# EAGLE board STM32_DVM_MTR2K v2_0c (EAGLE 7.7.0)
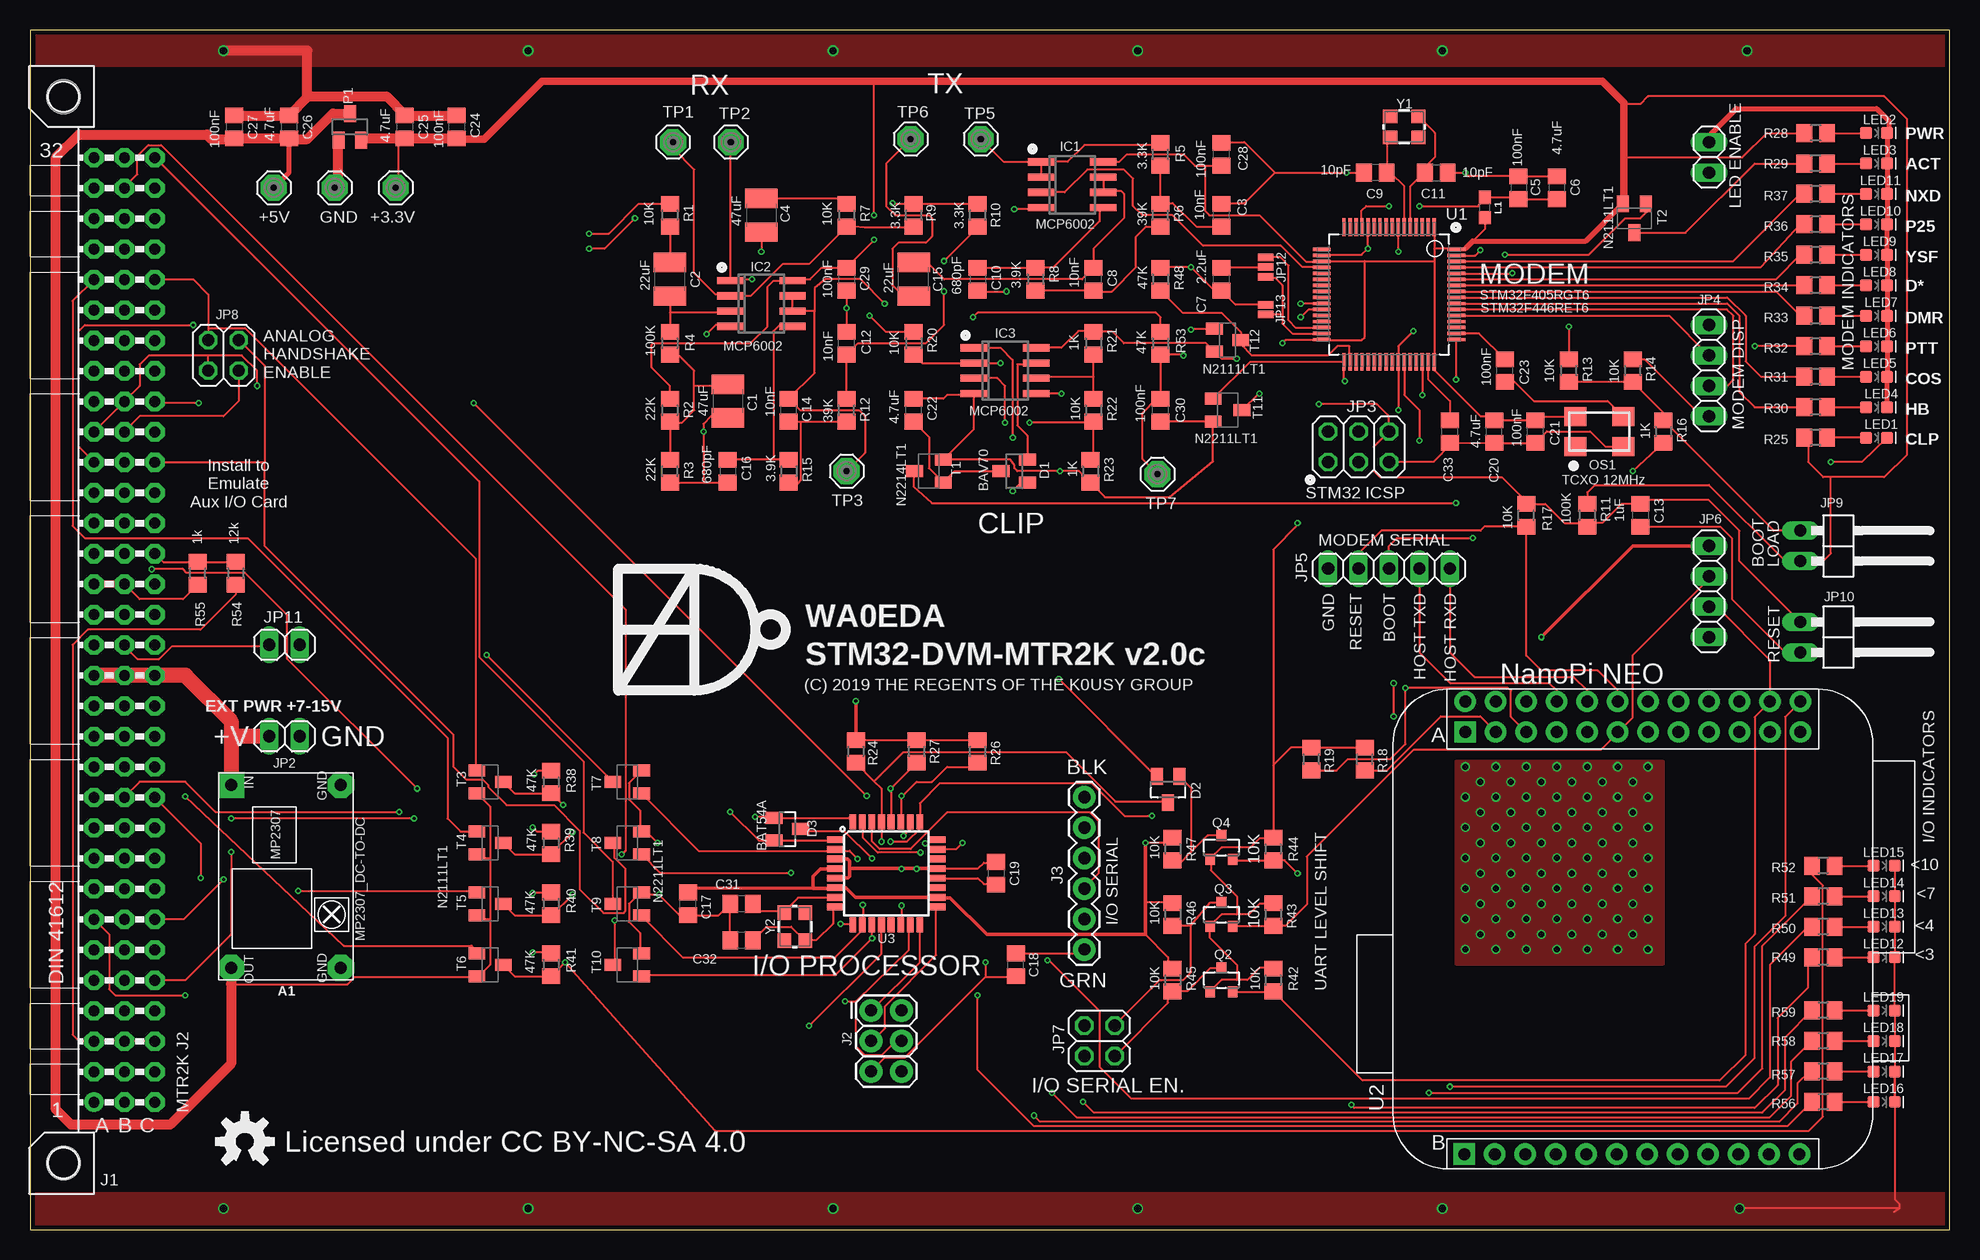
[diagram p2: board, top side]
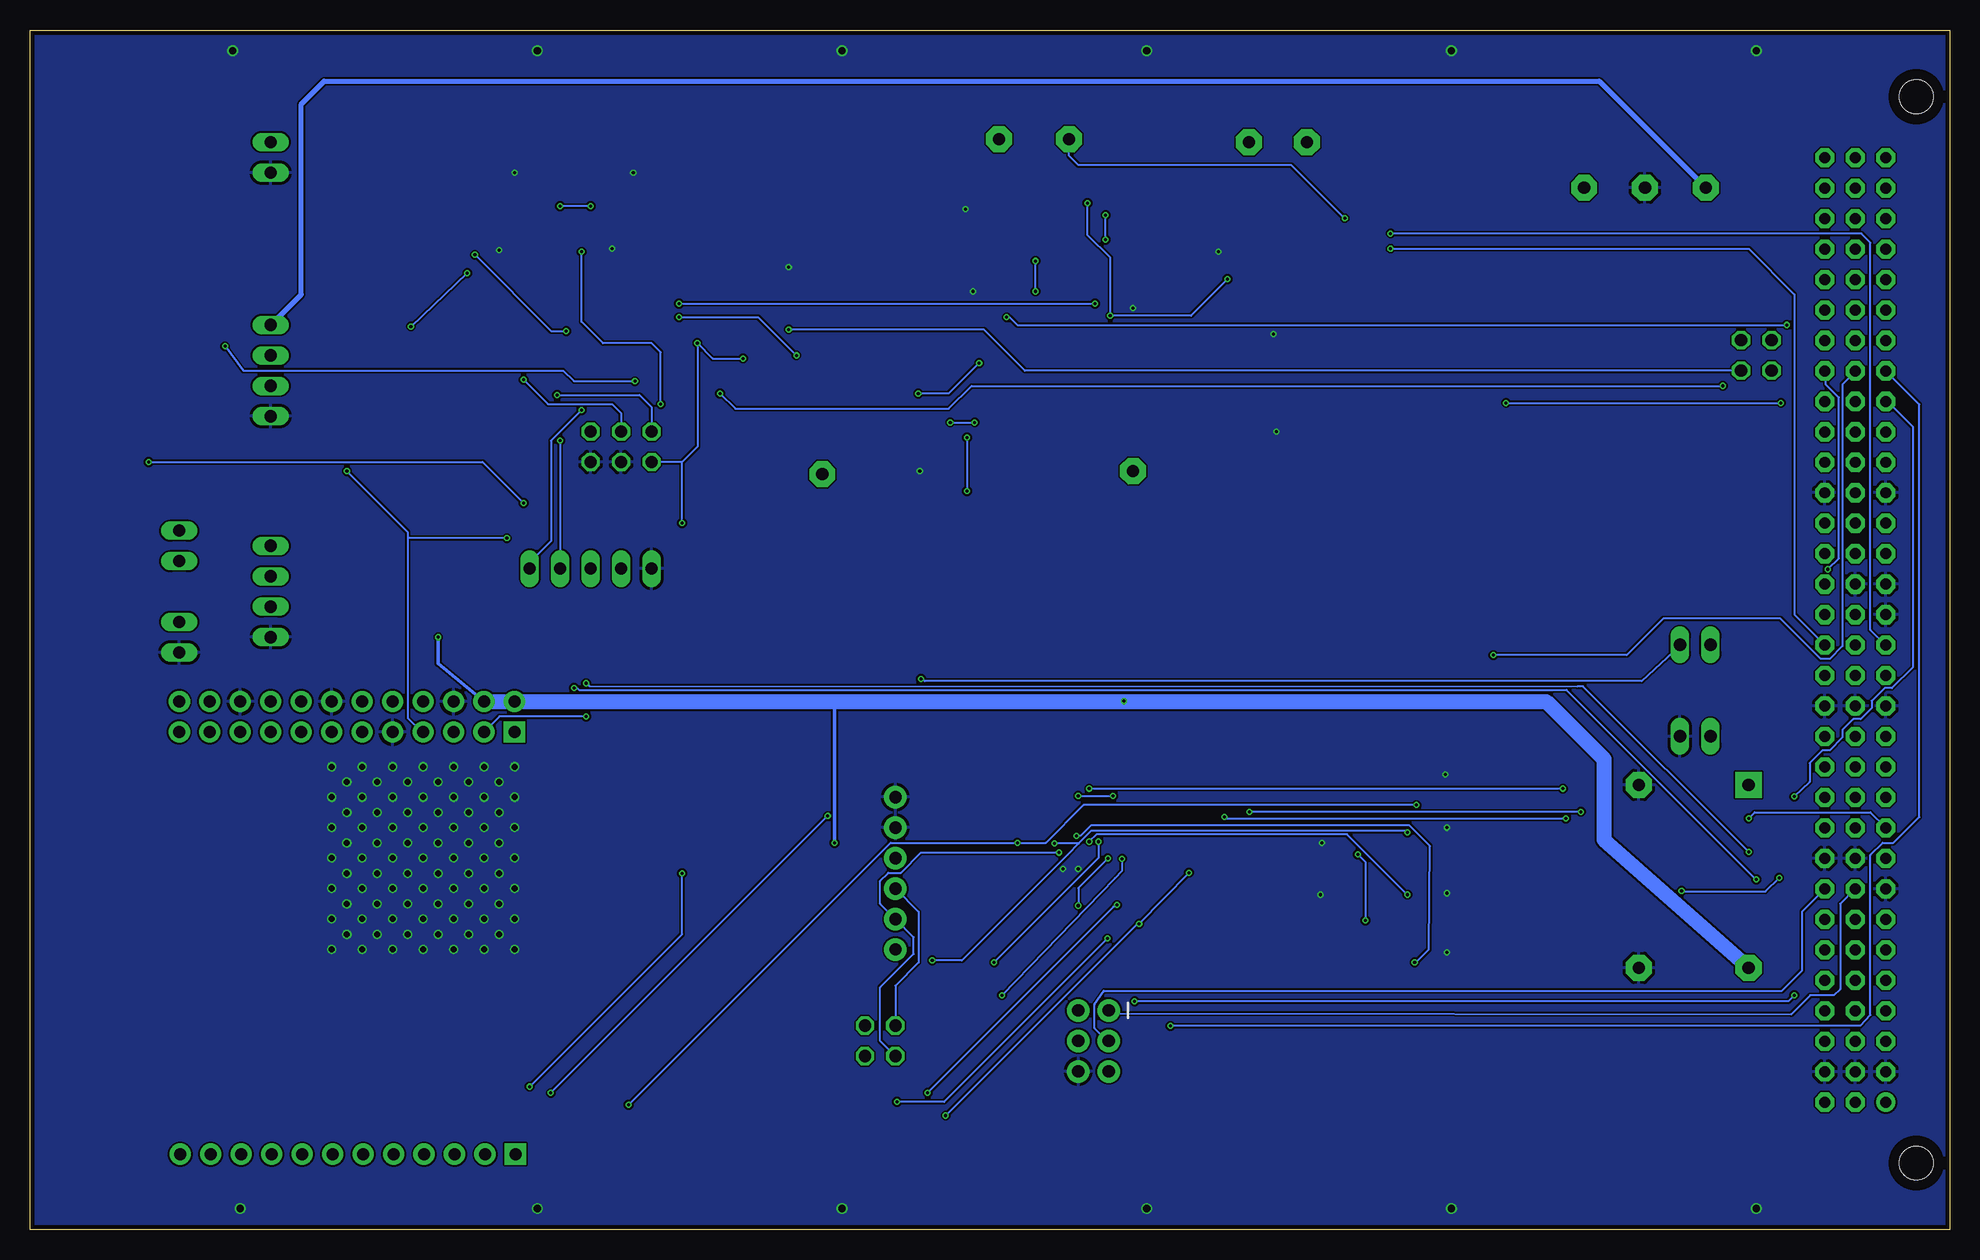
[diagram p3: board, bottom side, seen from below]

Size 160.02 x 100.03 mm. Coordinates in mm from the lower left corner, seen from the top.
Copper layers (1*16): Top 0.035559375mm / dielectric 1.6mm / Bottom 0.035559375mm
Design rules "oshpark-2layer-tented": minimum track width 6mil, minimum drill 10mil, track to track 6mil, track to pad 6mil, pad to pad 6mil, via to via 6mil, smd to smd 6mil, copper to edge 15mil, drill to drill 6mil, minimum pad ring 5mil, minimum via ring 5mil, stop-mask expansion 2.5mil, vias tented up to drill 20mil, thermal gap 10mil

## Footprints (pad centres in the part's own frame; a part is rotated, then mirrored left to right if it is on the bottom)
MCS10B = drill 1.016 pad 2.159 octagon: MP 0,0
MPS2307_DC-TO-DC = drill 1.016 pad 2.184 octagon: GND1 -7.62,4.572; GND2 7.62,4.572; OUT 7.62,-4.572 | drill 1.016 pad 2.184 square: IN -7.62,-4.572
C1210 = smd 1.6 x 2.7: 1 -1.4,0; 2 1.4,0
C0805 = smd 1.3 x 1.5: 1 -0.95,0; 2 0.95,0
SOT23C = smd 1 x 1.4: 1 -0.95,-1.1; 2 0.95,-1.1; 3 0,1.1
SOT23 = smd 1 x 1.4: 1 -0.95,-1.1; 2 0.95,-1.1; 3 0,1.1
SO08 = smd 0.6 x 2.2: 1 -1.905,-2.6; 2 -0.635,-2.6; 3 0.635,-2.6; 4 1.905,-2.6; 5 1.905,2.6; 6 0.635,2.6; 7 -0.635,2.6; 8 -1.905,2.6
VG96 = drill 0.914 pad 1.6: A1 154.94,39.37 | drill 0.914 pad 1.6 octagon: A2 154.94,36.83; A3 154.94,34.29; A4 154.94,31.75; A5 154.94,29.21; A6 154.94,26.67; A7 154.94,24.13; A8 154.94,21.59; A9 154.94,19.05; A10 154.94,16.51; A11 154.94,13.97; A12 154.94,11.43; A13 154.94,8.89; A14 154.94,6.35; A15 154.94,3.81; A16 154.94,1.27; A17 154.94,-1.27; A18 154.94,-3.81; A19 154.94,-6.35; A20 154.94,-8.89; A21 154.94,-11.43; A22 154.94,-13.97; A23 154.94,-16.51; A24 154.94,-19.05; A25 154.94,-21.59; A26 154.94,-24.13; A27 154.94,-26.67; A28 154.94,-29.21; A29 154.94,-31.75; A30 154.94,-34.29; A31 154.94,-36.83; A32 154.94,-39.37; B1 152.4,39.37; B2 152.4,36.83; B3 152.4,34.29; B4 152.4,31.75; B5 152.4,29.21; B6 152.4,26.67; B7 152.4,24.13; B8 152.4,21.59; B9 152.4,19.05; B10 152.4,16.51; B11 152.4,13.97; B12 152.4,11.43; B13 152.4,8.89; B14 152.4,6.35; B15 152.4,3.81; B16 152.4,1.27; B17 152.4,-1.27; B18 152.4,-3.81; B19 152.4,-6.35; B20 152.4,-8.89; B21 152.4,-11.43; B22 152.4,-13.97; B23 152.4,-16.51; B24 152.4,-19.05; B25 152.4,-21.59; B26 152.4,-24.13; B27 152.4,-26.67; B28 152.4,-29.21; B29 152.4,-31.75; B30 152.4,-34.29; B31 152.4,-36.83; B32 152.4,-39.37; C1 149.86,39.37; C2 149.86,36.83; C3 149.86,34.29; C4 149.86,31.75; C5 149.86,29.21; C6 149.86,26.67; C7 149.86,24.13; C8 149.86,21.59; C9 149.86,19.05; C10 149.86,16.51; C11 149.86,13.97; C12 149.86,11.43; C13 149.86,8.89; C14 149.86,6.35; C15 149.86,3.81; C16 149.86,1.27; C17 149.86,-1.27; C18 149.86,-3.81; C19 149.86,-6.35; C20 149.86,-8.89; C21 149.86,-11.43; C22 149.86,-13.97; C23 149.86,-16.51; C24 149.86,-19.05; C25 149.86,-21.59; C26 149.86,-24.13; C27 149.86,-26.67; C28 149.86,-29.21; C29 149.86,-31.75; C30 149.86,-34.29; C31 149.86,-36.83; C32 149.86,-39.37 | hole 2.794: 157.48,44.45; 157.48,-44.45
2X3 = drill 1.016 pad 1.88: 1 0,0; 2 0,2.54; 3 2.54,0; 4 2.54,2.54; 5 5.08,0; 6 5.08,2.54
FTDI_BASIC = drill 1.016 pad 1.88: CTS 10.16,0; DTR 0,0; GND 12.7,0; RXI 2.54,0; TXO 5.08,0; VCC 7.62,0
1X02 = drill 1.016 long: 1 -1.27,0; 2 1.27,0
2X03 = drill 1.016 octagon: 1 -2.54,-1.27; 2 -2.54,1.27; 3 0,-1.27; 4 0,1.27; 5 2.54,-1.27; 6 2.54,1.27
1X04 = drill 1.016 long: 1 -3.81,0; 2 -1.27,0; 3 1.27,0; 4 3.81,0
1X05 = drill 1.016 long: 1 -5.08,0; 2 -2.54,0; 3 0,0; 4 2.54,0; 5 5.08,0
2X02 = drill 1.016 octagon: 1 -1.27,-1.27; 2 -1.27,1.27; 3 1.27,-1.27; 4 1.27,1.27
1X02/90 = drill 1.016 long: 1 -1.27,-3.81; 2 1.27,-3.81
SMT-JUMPER_3_NO_NO-SILK = smd 0.635 x 1.27: 1 -0.813,0; 2 0,0; 3 0.813,0
SMT-JUMPER_2_NO_NO-SILK = smd 0.635 x 1.27: 1 -0.406,0; 2 0.406,0
0603 = smd 1.1 x 1: 1 -0.85,0; 2 0.85,0
LED-0603 = smd 1 x 1: A -0.877,0; C 0.877,0
5.2X3.4-4-PAD = smd 1.8 x 1.6: 1 -2,-1.25; 2 2,-1.25; 3 2,1.25; 4 -2,1.25
XC6206_SOT-23 = smd 1 x 1.4: 1 -0.95,-1.1; 2 0.95,-1.1; 3 0,1.1
SOT23' = smd 0.8 x 0.9: 1 -0.95,-1; 2 0.95,-1; 3 0,1
R0805 = smd 1.3 x 1.5: 1 -0.95,0; 2 0.95,0
SC59-BEC = smd 1 x 1.4: B -0.95,-1.2; C 0,1.2; E 0.95,-1.2
SOT23-BEC = smd 1 x 1.4: B -0.95,-1.1; C 0,1.1; E 0.95,-1.1
QFP50P1200X1200X160-64N = smd 1.473 x 0.279: 1 -5.613,3.759; 2 -5.613,3.251; 3 -5.613,2.743; 4 -5.613,2.261; 5 -5.613,1.753; 6 -5.613,1.245; 7 -5.613,0.762; 8 -5.613,0.254; 9 -5.613,-0.254; 10 -5.613,-0.762; 11 -5.613,-1.245; 12 -5.613,-1.753; 13 -5.613,-2.261; 14 -5.613,-2.743; 15 -5.613,-3.251; 16 -5.613,-3.759; 33 5.613,-3.759; 34 5.613,-3.251; 35 5.613,-2.743; 36 5.613,-2.261; 37 5.613,-1.753; 38 5.613,-1.245; 39 5.613,-0.762; 40 5.613,-0.254; 41 5.613,0.254; 42 5.613,0.762; 43 5.613,1.245; 44 5.613,1.753; 45 5.613,2.261; 46 5.613,2.743; 47 5.613,3.251; 48 5.613,3.759 | smd 0.279 x 1.473: 17 -3.759,-5.613; 18 -3.251,-5.613; 19 -2.743,-5.613; 20 -2.261,-5.613; 21 -1.753,-5.613; 22 -1.245,-5.613; 23 -0.762,-5.613; 24 -0.254,-5.613; 25 0.254,-5.613; 26 0.762,-5.613; 27 1.245,-5.613; 28 1.753,-5.613; 29 2.261,-5.613; 30 2.743,-5.613; 31 3.251,-5.613; 32 3.759,-5.613; 49 3.759,5.613; 50 3.251,5.613; 51 2.743,5.613; 52 2.261,5.613; 53 1.753,5.613; 54 1.245,5.613; 55 0.762,5.613; 56 0.254,5.613; 57 -0.254,5.613; 58 -0.762,5.613; 59 -1.245,5.613; 60 -1.753,5.613; 61 -2.261,5.613; 62 -2.743,5.613; 63 -3.251,5.613; 64 -3.759,5.613
NANOPI-NEO = drill 1 pad 1.778 square: A1 6.02,36.42; B1 5.94,1.227 | drill 1 pad 1.778: A2 6.02,38.96; A3 8.56,36.42; A4 8.56,38.96; A5 11.1,36.42; A6 11.1,38.96; A7 13.64,36.42; A8 13.64,38.96; A9 16.18,36.42; A10 16.18,38.96; A11 18.72,36.42; A12 18.72,38.96; A13 21.26,36.42; A14 21.26,38.96; A15 23.8,36.42; A16 23.8,38.96; A17 26.34,36.42; A18 26.34,38.96; A19 28.88,36.42; A20 28.88,38.96; A21 31.42,36.42; A22 31.42,38.96; A23 33.96,36.42; A24 33.96,38.96; B2 8.48,1.227; B3 11.02,1.227; B4 13.56,1.227; B5 16.1,1.227; B6 18.64,1.227; B7 21.18,1.227; B8 23.72,1.227; B9 26.26,1.227; B10 28.8,1.227; B11 31.34,1.227; B12 33.88,1.227
TQFP32-08 = smd 1.27 x 0.559: 1 -4.293,2.8; 2 -4.293,2; 3 -4.293,1.2; 4 -4.293,0.4; 5 -4.293,-0.4; 6 -4.293,-1.2; 7 -4.293,-2; 8 -4.293,-2.8; 17 4.293,-2.8; 18 4.293,-2; 19 4.293,-1.2; 20 4.293,-0.4; 21 4.293,0.4; 22 4.293,1.2; 23 4.293,2; 24 4.293,2.8 | smd 0.559 x 1.27: 9 -2.8,-4.293; 10 -2,-4.293; 11 -1.2,-4.293; 12 -0.4,-4.293; 13 0.4,-4.293; 14 1.2,-4.293; 15 2,-4.293; 16 2.8,-4.293; 25 2.8,4.293; 26 2,4.293; 27 1.2,4.293; 28 0.4,4.293; 29 -0.4,4.293; 30 -1.2,4.293; 31 -2,4.293; 32 -2.8,4.293
CRYSTAL-SMD-3.2X2.5MM = smd 1.2 x 1.1: 1 -1.175,-0.875; 2 1.175,-0.875; 3 1.175,0.875; 4 -1.175,0.875

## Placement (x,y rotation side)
+3.3V  MCS10B  [MCS10B]  30.48,86.87 0 top
+5V  MCS10B  [MCS10B]  20.32,86.87 0 top
A1  MP2307_DC-TO-DC  [MPS2307_DC-TO-DC]  21.34,29.46 270 top
C1  47uF  [C1210]  58.17,69.09 270 top
C2  22uF  [C1210]  53.34,79.25 90 top
C3  10nF  [C0805]  99.31,84.58 90 top
C4  47uF  [C1210]  60.96,84.58 270 top
C5  100nF  [C0805]  124.08,86.87 270 top
C6  4.7uF  [C0805]  127.25,86.87 270 top
C7  2.2uF  [C0805]  99.31,79.25 90 top
C8  10nF  [C0805]  88.65,79.25 90 top
C9  10pF  [C0805]  112.14,88.14 180 top
C10  680pF  [C0805]  78.99,79.25 270 top
C11  10pF  [C0805]  117.22,88.14 0 top
C12  10nF  [C0805]  68.07,73.91 90 top
C13  1uF  [C0805]  134.24,59.56 270 top
C14  10nF  [C0805]  63.25,68.33 90 top
C15  22uF  [C1210]  73.66,79.25 90 top
C16  680pF  [C0805]  58.17,63.25 270 top
C17  100nF  [C0805]  54.86,27.18 90 top
C18  100nF  [C0805]  82.17,22.1 90 top
C19  100nF  [C0805]  80.52,29.72 270 top
C20  4.7uF  [C0805]  122.05,66.55 90 top
C21  100nF  [C0805]  125.48,66.55 90 top
C22  4.7uF  [C0805]  73.66,68.33 90 top
C23  100nF  [C0805]  122.94,71.63 90 top
C24  100nF  [C0805]  35.56,91.95 270 top
C25  4.7uF  [C0805]  31.24,91.95 270 top
C26  4.7uF  [C0805]  21.59,91.95 270 top
C27  100nF  [C0805]  17.02,91.95 270 top
C28  100nF  [C0805]  99.31,89.66 90 top
C29  100nF  [C0805]  68.07,79.25 270 top
C30  100nF  [C0805]  94.23,68.33 90 top
C31  10pF  [C0805]  59.31,27.18 180 top
C32  10pF  [C0805]  59.31,24.13 180 top
C33  2.2uF  [C0805]  118.36,66.55 90 top
D1  BAV70  [SOT23C]  82.04,63.25 90 top
D2  BAT54A  [SOT23]  94.87,36.7 180 top
D3  BAT54A  [SOT23]  63.12,33.4 270 top
GND  MCS10B  [MCS10B]  25.4,86.87 0 top
IC1  MCP6002  [SO08]  86.87,87.12 270 top
IC2  MCP6002  [SO08]  60.96,77.22 270 top
IC3  MCP6002  [SO08]  81.28,71.63 270 top
J1  MTR2K J2  [VG96]  160.27,50.01 180 top
J2  AVR_SPI_ICSP  [2X3]  70.1,18.29 270 top
J3  I/O SERIAL  [FTDI_BASIC]  87.88,23.37 90 top
JP1  LED ENABLE  [1X02]  139.95,89.41 270 top
JP2  EXT PWR +7-15V  [1X02]  21.21,41.15 0 top
JP3  STM32 ICSP  [2X03]  110.74,65.28 0 top
JP4  MODEM DISP  [1X04]  139.95,71.63 270 top
JP5  MODEM SERIAL  [1X05]  113.28,55.12 180 top
JP6  SBC DISP  [1X04]  139.95,53.21 270 top
JP7  I/O SERIAL EN.  [2X02]  89.15,15.75 90 top
JP8  ANALOG HANDSHAKE ENABLE  [2X02]  16.13,72.9 180 top
JP9  BOOT  [1X02/90]  151.38,57.02 270 top
JP10  RESET  [1X02/90]  151.38,49.4 270 top
JP11  AVR RESET  [1X02]  21.21,48.77 0 top
JP12  405/446  [SMT-JUMPER_3_NO_NO-SILK]  103,80.26 270 top
JP13  446  [SMT-JUMPER_2_NO_NO-SILK]  103,76.71 90 top
L1  120Ω/100M  [0603]  121.28,85.22 90 top
LED1  RED  [LED-0603]  153.92,66.04 0 top
LED2  BLU  [LED-0603]  153.92,91.44 0 top
LED3  ORG  [LED-0603]  153.92,88.9 0 top
LED4  ORG  [LED-0603]  153.92,68.58 0 top
LED5  GRN  [LED-0603]  153.92,71.12 0 top
LED6  RED  [LED-0603]  153.92,73.66 0 top
LED7  YEL  [LED-0603]  153.92,76.2 0 top
LED8  YEL  [LED-0603]  153.92,78.74 0 top
LED9  YEL  [LED-0603]  153.92,81.28 0 top
LED10  YEL  [LED-0603]  153.92,83.82 0 top
LED11  YEL  [LED-0603]  153.92,86.36 0 top
LED12  GRN  [LED-0603]  154.56,22.73 0 top
LED13  GRN  [LED-0603]  154.56,25.27 0 top
LED14  GRN  [LED-0603]  154.56,27.81 0 top
LED15  GRN  [LED-0603]  154.56,30.35 0 top
LED16  RED  [LED-0603]  154.56,10.67 0 top
LED17  RED  [LED-0603]  154.56,13.21 0 top
LED18  RED  [LED-0603]  154.56,15.75 0 top
LED19  RED  [LED-0603]  154.56,18.29 0 top
OS1  TCXO 12MHz  [5.2X3.4-4-PAD]  130.81,66.55 0 top
P1  XC6206P332MR  [XC6206_SOT-23]  26.67,91.95 0 top
Q2  BSS138  [SOT23']  99.31,20.83 0 top
Q3  BSS138  [SOT23']  99.31,26.29 0 top
Q4  BSS138  [SOT23']  99.31,31.88 0 top
R1  10K  [R0805]  53.34,84.58 270 top
R2  22K  [R0805]  53.34,68.33 270 top
R3  22K  [R0805]  53.34,63.25 90 top
R4  100K  [R0805]  53.34,73.91 270 top
R5  3.3K  [R0805]  94.23,89.66 90 top
R6  39K  [R0805]  94.23,84.58 90 top
R7  10K  [R0805]  68.07,84.58 270 top
R8  3.9K  [R0805]  83.82,79.25 270 top
R9  3.3K  [R0805]  73.66,84.58 90 top
R10  3.3K  [R0805]  78.99,84.58 90 top
R11  100K  [R0805]  129.79,59.56 270 top
R12  39K  [R0805]  68.07,68.33 90 top
R13  10K  [R0805]  128.27,71.63 90 top
R14  10K  [R0805]  133.6,71.63 90 top
R15  3.9K  [R0805]  63.25,63.25 270 top
R16  1K  [R0805]  136.14,66.55 270 top
R17  10K  [R0805]  124.71,59.56 90 top
R18  3.3K  [R0805]  111.25,39.24 90 top
R19  3.3K  [R0805]  106.81,39.24 90 top
R20  10K  [R0805]  73.66,73.91 270 top
R21  1K  [R0805]  88.65,73.91 270 top
R22  10K  [R0805]  88.65,68.33 270 top
R23  1K  [R0805]  88.39,63.25 270 top
R24  10K  [R0805]  68.83,39.88 270 top
R25  560  [R0805]  148.84,66.04 180 top
R26  3.3K  [R0805]  78.99,39.88 90 top
R27  3.3K  [R0805]  73.91,39.88 90 top
R28  1K  [R0805]  148.84,91.44 180 top
R29  560  [R0805]  148.84,88.9 180 top
R30  560  [R0805]  148.84,68.58 180 top
R31  1K  [R0805]  148.84,71.12 180 top
R32  560  [R0805]  148.84,73.66 180 top
R33  560  [R0805]  148.84,76.2 180 top
R34  560  [R0805]  148.84,78.74 180 top
R35  560  [R0805]  148.84,81.28 180 top
R36  560  [R0805]  148.84,83.82 180 top
R37  560  [R0805]  148.84,86.36 180 top
R38  47K  [R0805]  43.43,37.34 270 top
R39  47K  [R0805]  43.43,32.26 270 top
R40  47K  [R0805]  43.43,27.18 270 top
R41  47K  [R0805]  43.43,22.1 270 top
R42  10K  [R0805]  103.63,20.83 270 top
R43  10K  [R0805]  103.63,26.29 270 top
R44  10K  [R0805]  103.63,31.75 270 top
R45  10K  [R0805]  95.25,20.83 270 top
R46  10K  [R0805]  95.25,26.29 270 top
R47  10K  [R0805]  95.25,31.75 270 top
R48  47K  [R0805]  94.23,79.25 270 top
R49  1K  [R0805]  149.48,22.73 180 top
R50  1K  [R0805]  149.48,25.27 180 top
R51  1K  [R0805]  149.48,27.81 180 top
R52  1K  [R0805]  149.48,30.35 180 top
R53  47K  [R0805]  94.23,73.91 270 top
R54  12k  [R0805]  17.14,54.74 270 top
R55  1k  [R0805]  13.97,54.74 90 top
R56  1K  [R0805]  149.48,10.67 180 top
R57  1K  [R0805]  149.48,13.21 180 top
R58  1K  [R0805]  149.48,15.75 180 top
R59  1K  [R0805]  149.48,18.29 180 top
T1  N2214LT1  [SC59-BEC]  74.93,63.25 90 top
T2  N2111LT1  [SC59-BEC]  133.73,84.33 180 top
T3  N2111LT1  [SOT23-BEC]  38.35,37.34 270 top
T4  N2111LT1  [SOT23-BEC]  38.35,32.26 270 top
T5  N2111LT1  [SOT23-BEC]  38.35,27.18 270 top
T6  N2111LT1  [SOT23-BEC]  38.35,22.1 270 top
T7  N2211LT1  [SC59-BEC]  49.78,37.34 90 top
T8  N2211LT1  [SC59-BEC]  49.78,32.26 90 top
T9  N2211LT1  [SC59-BEC]  49.78,27.18 90 top
T10  N2211LT1  [SC59-BEC]  49.78,22.1 90 top
T11  N2211LT1  [SC59-BEC]  99.82,68.33 270 top
T12  N2111LT1  [SOT23-BEC]  99.82,74.17 270 top
TP1  MCS10B  [MCS10B]  53.59,90.68 0 top
TP2  MCS10B  [MCS10B]  58.42,90.68 0 top
TP3  MCS10B  [MCS10B]  68.07,63.25 0 top
TP5  MCS10B  [MCS10B]  79.25,90.93 0 top
TP6  MCS10B  [MCS10B]  73.41,90.93 0 top
TP7  MCS10B  [MCS10B]  93.98,62.99 0 top
U1  STM32F405RGT6  [QFP50P1200X1200X160-64N]  113.28,77.98 270 top
U2  NanoPi NEO  [NANOPI-NEO]  113.61,5.08 0 top
U3  ATMEGA328P_TQFP  [TQFP32-08]  71.37,29.72 0 top
U$1  [EDA]  49.02,44.96 0 top
U$2  [OSHW-LOGO-M]  17.91,7.37 0 top
Y1  8MHz  [CRYSTAL-SMD-3.2X2.5MM]  114.55,91.95 0 top
Y2  16MHz  [CRYSTAL-SMD-3.2X2.5MM]  63.75,25.27 90 top

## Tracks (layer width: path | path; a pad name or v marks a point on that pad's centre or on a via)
14.2V
  Top 1.27: J1.A15 J1.B15 J1.C15 10.44,46.23 12.95,46.23 | 12.98,46.23 12.95,46.23 | 12.95,46.23 16.76,42.42 16.76,41.15 | 16.76,41.15 A1.IN | JP2.1 16.76,41.15
  Bottom 1.422: J1.C15 10.44,46.23
+3V3  (via drill 0.25)
  Top 0.152: OS1.4 125.78,67.8 C21.2 C20.2 121.73,67.82 120.9,67.82 117.09,71.63 117.09,72.31 U1.48 117.04,80.77 | U1.64 118.95,81.79 | 118.95,81.79 119.63,81.79 | 132.84,89.41 142.75,89.41 144.78,91.44 R28.2 | U1.1 117.04,81.79 | 117.04,81.79 117.04,80.77 | 118.95,81.79 117.04,81.79 | 111.25,80.77 107.72,80.77 107.7,80.82 U1.19 106.35,80.72 102.49,84.58 98.3,84.58 97.92,84.96 97.92,88.71 | 111.25,80.77 117.04,80.77 | 111.25,80.77 111.25,74.42 111,74.17 107.72,74.17 U1.32 107.62,74.17 104.65,74.17 v104.39,73.91 | v70.36,82.55 70.36,82.48 C29.1 65.97,80.2 65.02,79.25 63.69,79.25 IC2.8 61.98,79.12 61.47,78.61 61.47,75.31 60.07,73.91 51.94,73.91 51.82,73.79 51.82,71.88 53.34,70.36 R2.1 | v70.36,84.58 70.36,95.76 | IC3.8 85.98,73.53 87.38,74.93 88.58,74.93 R21.1 90.24,74.86 91.19,73.91 98.03,73.91 T12.E 99.3,72.64 v100.58,72.64 | 132.84,93.85 134.24,93.85 134.87,94.49 154.56,94.49 156.46,92.58 156.46,64.64 154.56,62.74 150.11,62.74 | R25.2 148.21,65.72 148.21,64.01 149.48,62.74 150.11,62.74 | IC1.8 90.8,89.03 91.44,89.66 96.14,89.66 97.09,88.71 97.92,88.71 | 97.92,88.71 C28.1 | R42.1 103.57,21.84 102.49,21.84 101.47,20.83 100.58,20.83 | 100.58,20.83 99.31,20.83 98.36,19.88 Q2.1 | R43.1 103.57,27.18 102.49,27.18 101.6,26.29 100.58,26.29 | 100.58,26.29 99.31,26.29 98.36,25.34 Q3.1 98.36,24.32 100.58,22.1 100.58,20.83 | 100.58,26.29 100.58,27.81 98.42,29.97 98.42,30.82 Q4.1 98.36,30.93 99.31,31.88 101.73,31.88 102.49,32.64 103.57,32.64 R44.1 103.63,38.73 | v105.66,58.93 105.66,58.73 103.63,56.7 103.63,38.73 | 35.61,91.03 35.63,90.93 | +3.3V.MP 30.73,87.12 30.73,91 | R11.1 129.79,61.47 130.43,62.1 139.95,62.1 146.3,55.75 JP9.2 149.48,55.75 150.11,56.39 150.11,62.74
  Top 0.152: 103.63,38.73 105.09,40.19 R19.2 R18.2 | 120.61,82.42 120.27,82.42 121.28,83.44 L1.1
  Top 0.406: 119.63,81.79 120.27,82.42 129.68,82.42 T2.E
  Top 0.61: 35.63,90.93 37.85,90.93 42.67,95.76 70.36,95.76 131.06,95.76 132.84,93.98 132.84,93.85 132.84,89.41 132.84,85.59 T2.E
  Top 0.813: P1.2 27.77,91 30.73,91 C25.2 C24.2 35.6,91.03 35.61,91.03
  Bottom 0.152: v70.36,82.55 v70.36,84.58 | 105.66,64.01 104.39,65.28 v104.39,73.91 103.12,72.64 v100.58,72.64 | 105.66,64.01 JP3.1 | v105.66,58.93 105.66,64.01
+5V  (via drill 0.25)
  Top 0.152: 94.93,21.46 R45.1 94.87,22.16 94.87,22.73 92.96,24.64 | R46.1 95.19,27.18 95.06,27.3 92.96,27.3 | U3.18 75.7,27.69 | R47.1 94.81,32.26 v92.96,32.26 | R24.1 R27.2 R26.2 | T3.E 38.35,35.29 38.35,30.99 | 38.35,30.99 38.35,25.91 | 38.35,25.91 38.35,22.1 37.4,21.15 T6.E 37.13,21.08 27.08,21.08 26.47,20.47 16.76,20.47 | T4.E 37.57,30.99 38.35,30.99 | T5.E 37.57,25.91 38.35,25.91
  Top 0.254: 65.28,28.45 54.86,28.45 C17.2
  Top 0.305: v92.96,32.26 92.96,27.3 92.96,24.64 79.76,24.64 76.71,27.69 75.7,27.69 | JP6.1 133.6,57.02 v125.98,49.4 | U3.18 68.8,27.72 68,28.52 U3.6 67.01,28.45 65.28,28.45 65.28,29.46 65.91,30.1 67.06,30.1 U3.4 | R24.1 v68.83,44.07
  Top 0.406: C26.2 21.59,88.14 +5V.MP
  Top 0.813: A1.OUT 16.76,20.47 16.76,13.84 11.68,8.76 3.43,8.76 2.16,10.03 2.16,89.41 4.06,91.31 14.73,91.31 15.11,90.93 16.95,90.93 C27.2 C26.2 21.66,90.93 23.11,90.93 25.23,93.05 P1.3
  Bottom 0.305: v125.98,49.4 125.98,47.21 U2.A4 | v92.96,32.26 92.96,44.04 | v68.83,44.07 68.83,44.04
  Bottom 0.406: JP4.1 137.41,77.98 137.41,93.85 135.51,95.76 29.21,95.76 +5V.MP
  Bottom 1.27: U2.A4 U2.A2 92.96,44.04 68.83,44.04 33.63,44.04 28.83,39.24 28.83,32.51 A1.OUT
AREF
  Top 0.152: U3.20 75.69,29.31 79.02,29.31 79.5,28.83 80.46,28.83 C19.2
AVR_PROG
  Top 0.152: D2.1 96.77,36.85 96.77,31.5 | 96.77,31.5 95.76,30.48 | Q4.3 98.15,32.88 96.77,31.5
  Top 0.305: 95.76,30.48 95.57,30.48 R47.2
AVR_RESET  (via drill 0.25)
  Top 0.152: v85.75,45.92 93.83,37.85 D2.2
  Bottom 0.152: v85.75,45.92 85.45,45.74 25.68,45.74 22.5,48.67 JP11.2
AVR_RX
  Top 0.152: R46.2 95.31,25.4 96.77,25.4 | 96.77,25.4 98.41,27.29 Q3.3 | 94.23,20.83 94.28,20.83 | 94.28,20.83 96.14,20.83 96.77,21.46 96.77,25.4 | JP7.3 90.47,17.12 94.13,20.78 94.28,20.78 94.28,20.83
AVR_SCL  (via drill 0.25)
  Top 0.152: R27.1 71.77,36.79 71.77,36.78 | 71.77,36.78 U3.28 | v10.16,55.07 12.75,55.07 13.06,54.76 17.93,54.76 21.44,51.26 21.44,47.6 v32.26,36.78 | v71.73,36.78 71.77,36.78
  Bottom 0.152: v10.16,55.07 9.25,55.98 9.25,69.39 10.31,70.46 10.31,71.53 J1.C25 | v71.73,36.78 v32.26,36.78
AVR_SDA  (via drill 0.25)
  Top 0.152: U3.27 72.64,34.08 72.64,36.07 72.69,36.12 | 72.69,36.12 73.91,37.34 75.18,37.34 76.45,38.61 78.99,38.61 R26.1 | v14.07,68.94 10.46,68.94 J1.C24 | v69.75,36.17 v36.98,68.94 | v72.64,36.17 72.69,36.12
  Bottom 0.152: v36.98,68.94 v14.07,68.94 | v72.64,36.17 v69.75,36.17
AVR_TX
  Top 0.152: Q2.3 98.41,21.83 96.52,19.94 95.31,19.94 R45.2 94.87,19.5 94.87,18.95 | 94.87,18.92 94.87,18.95 | JP7.1 94.89,18.95 94.87,18.95
BOOT  (via drill 0.25)
  Top 0.152: R16.2 v133.6,63.25 | JP5.3 113.28,57.02 113.92,57.66 v120.27,57.66
  Bottom 0.152: v133.6,63.25 128.52,58.17 128.52,57.66 | 128.52,57.66 128.52,42.67 127.35,41.5 U2.A7 | v120.27,57.66 128.52,57.66
BOOT0  (via drill 0.25)
  Top 0.152: U1.60 123.42,79.73 v123.57,79.76 | v128.27,75.31 R13.2
  Bottom 0.152: v123.57,79.76 v128.27,75.31
CS1  (via drill 0.25)
  Top 0.152: D3.2 67.01,32.45 U3.1 | v30.76,34.85 15.44,34.85 12.95,37.34 9.14,37.34 7.87,36.07 J1.B11 | 61.98,32.51 D3.2 | v58.37,34.85 60.77,32.45 D3.2
  Bottom 0.152: v30.76,34.85 v58.37,34.85
CS2  (via drill 0.25)
  Top 0.152: U3.32 68.23,34.35 D3.1 61.95,34.42 v60.45,34.42 | v32,34.29 v16.76,34.29
  Bottom 0.152: v60.45,34.42 60.32,34.29 v32,34.29 | v16.76,34.29 16.26,34.8 6.6,34.8 5.33,33.53 J1.A10
DISP_RX
  Top 0.152: U1.54 141.45,76.73 141.99,76.2 141.99,70.87 141.48,70.36 JP4.3
DISP_TX
  Top 0.152: U1.53 118.92,76.2 136.65,76.2 JP4.2
DTR
  Top 0.152: C18.2 87.56,23.05 J3.DTR
EXT_CLK
  Top 0.152: C23.2 120.79,74.73 U1.50
GND  (via drill 0.25, 0.5, 0.6)
  Top 0.152: OS1.2 131.3,65.3 130.05,66.55 126.43,66.55 C21.1 C20.1 118.55,65.53 118.49,65.53 | 111.51,83.62 U1.12 111.53,82.07 v111.51,81.79 111,81.28 107.7,81.28 U1.18 107.54,81.28 | C22.2 76.13,69.28 76.45,69.6 78.55,69.6 IC3.4 78.68,66.75 T1.E 81.72,64.2 82.04,63.75 82.04,63.5 82.3,63.25 v85.85,63.25 87.44,63.25 R23.2 89.6,61.09 95,61.09 98.62,64.08 T11.E C30.1 | R48.1 93.79,80.2 93.73,80.26 v96.77,80.26 98.74,78.3 C7.1 100.5,77.11 JP13.2 | C12.2 v68.07,76.83 C29.2 68.01,78.23 | C10.2 79.06,78.23 v81.41,78.23 | IC1.4 84.14,85.09 v82.04,85.09 | C4.2 v60.96,81.53 | IC2.4 58.23,75.44 57.15,75.44 v56.39,74.68 | 118.49,65.53 116.97,64.01 JP3.5 | C28.2 99.38,90.68 101.22,90.68 103.76,88.14 | 103.76,88.14 v109.73,88.14 C9.2 | C3.2 99.38,85.6 101.22,85.6 103.76,88.14 | 56.13,62.3 R3.1 52.96,62.1 | 56.13,62.3 C16.2 | C1.2 58.04,67.82 56.77,67.82 56.13,67.18 v56.13,66.55 56.13,62.3 | R14.2 134.56,72.58 139.32,67.82 JP4.4 | v42.04,37.97 42.36,38.29 R38.1 | v41.91,33.53 42.23,33.21 R39.1 | R55.1 12.76,52.58 9.14,52.58 7.9,53.82 J1.B18 | LED16.C LED18.C LED19.C LED12.C LED13.C LED14.C LED15.C | LED16.C LED17.C | 155.35,1.49 155.83,1.78 | 155.83,1.78 v142.49,1.78 | C13.2 140.9,58.61 141.86,57.66 141.86,52.58 146.3,48.13 JP10.2 | 68.34,30.12 68.33,30.1 | v73.91,30.1 73.93,30.12 U3.21 79.01,30.12 79.5,30.61 80.46,30.61 C19.1 | R40.1 43.37,28.07 v41.91,28.07 | R41.1 43.37,23.11 v41.91,23.11 | T10.E 50.85,23.06 50.85,24.74 49.94,25.65 49.94,27.18 50.85,28.09 T9.E 51.17,27.94 v52.45,27.94 54.16,26.23 C17.1 57.41,26.23 C31.2 C32.2 | T7.E 50.85,38.15 49.94,37.24 49.94,35.86 50.85,34.95 50.85,33.27 T8.E 51.37,33.21 v52.32,32.26
  Top 0.152: C6.1 127.2,87.83 124.15,87.83 C5.1 119.95,87.82 v119.63,88.14 C11.2 | U1.63 120.47,81.23 v120.9,81.66 | C33.1 118.36,65.58 118.52,65.58 118.49,65.53 | LED16.C 155.45,10.66 155.45,2.54 155.83,2.16 155.83,1.78
  Top 0.305: U3.3 68.14,30.92 68.33,30.73 68.33,30.1 68.33,29.46 68.18,29.32 U3.5 | U3.21 68.34,30.12
  Top 0.61: J1.A18 J1.B18
  Top 0.813: P1.1 25.65,90.78 25.65,86.87 GND.MP | 23.18,94.49 C26.1 C27.1 | 23.18,94.49 29.72,94.49 31.24,92.96 C25.1 C24.1 | 23.18,94.49 23.11,94.55 23.11,98.3 v16.13,98.3
  other vias: 132.33,25.91 119.63,38.61 122.17,38.61 124.71,38.61 127.25,38.61 129.79,38.61 132.33,38.61 134.87,38.61 134.87,36.07 132.33,36.07 129.79,36.07 127.25,36.07 124.71,36.07 122.17,36.07 119.63,36.07 119.63,33.53 122.17,33.53 124.71,33.53 127.25,33.53 129.79,33.53 132.33,33.53 134.87,33.53 134.87,30.99 132.33,30.99 129.79,30.99 127.25,30.99 124.71,30.99 122.17,30.99 119.63,30.99 119.63,28.45 119.63,25.91 119.63,23.37 122.17,23.37 122.17,25.91 122.17,28.45 124.71,28.45 124.71,25.91 124.71,23.37 127.25,23.37 127.25,25.91 127.25,28.45 129.79,28.45 129.79,25.91 129.79,23.37 132.33,28.45 132.33,23.37 134.87,23.37 134.87,25.91 134.87,28.45 41.53,98.3 41.53,1.78 16.13,1.78 66.93,98.3 92.33,98.3 117.73,98.3 143.13,98.3 66.93,1.78 92.33,1.78 117.73,1.78 72.64,30.1 120.9,37.34 123.44,37.34 125.98,37.34 128.52,37.34 131.06,37.34 133.6,37.34 133.6,34.8 131.06,34.8 128.52,34.8 125.98,34.8 123.44,34.8 120.9,34.8 120.9,32.26 120.9,29.72 120.9,27.18 120.9,24.64 123.44,24.64 125.98,24.64 128.52,24.64 131.06,24.64 133.6,24.64 133.6,27.18 131.06,27.18 128.52,27.18 125.98,27.18 123.44,27.18 123.44,29.72 123.44,32.26 125.98,32.26 125.98,29.72 128.52,29.72 128.52,32.26 131.06,32.26 131.06,29.72 133.6,29.72 133.6,32.26
  pour Bottom: 0,0 160.02,0 160.02,100.03 0,99.95
  pour Top: 0.51,99.82 0.51,97.03 159.64,97.03 159.64,99.82
  pour Top: 0,0 160.02,0 160.02,3.05 0,3.05
  pour Top: 118.87,39.12 136.14,39.12 136.14,22.1 118.87,22.1
GPI_3
  Top 0.152: J1.C28 10.44,79.25 13.59,79.25 14.86,77.98 14.86,75.18 | 14.86,75.18 JP8.3 | 14.86,75.18 17.93,75.18 37.13,55.98 37.13,38.3 T3.B
GPI_4
  Top 0.152: J1.A28 3.56,77.44 3.56,58.67 4.57,57.66 18.16,57.66 34.8,41.02 34.8,34.29 35.88,33.21 T4.B
GPI_7  (via drill 0.25)
  Top 0.152: v22.35,28.24 37.13,28.24 T5.B | J1.C11 14.22,32.23 v14.22,29.34
  Bottom 0.152: v22.35,28.24 22.3,28.19 15.37,28.19 v14.22,29.34
GPI_10  (via drill 0.25)
  Top 0.152: 36.77,23.68 36.8,23.65 | 36.8,23.65 T6.B | v12.95,36.12 26.16,23.67 36.83,23.67 36.8,23.65
  Bottom 0.152: v12.95,36.12 11.68,37.34 11.68,38.91 10.62,39.98 10.01,39.98 8.94,41.05 8.94,41.66 8.03,42.57 7.42,42.57 6.5,43.48 6.5,44.09 5.44,45.16 4.83,45.16 3.05,46.94 3.05,66.93 5.18,69.06 J1.A24
GPO_0  (via drill 0.25)
  Top 0.152: v38.05,47.9 48.56,37.39 T7.C
  Bottom 0.152: v38.05,47.9 26.92,47.9 23.88,50.95 14.12,50.95 10.77,47.6 10.01,47.6 8.94,48.67 8.94,70.46 7.87,71.53 J1.B25
GPO_2
  Top 0.152: T8.C 48.72,32.21 48.72,30.99 49.63,30.07 49.63,26.57 49.48,26.42 47.8,26.42 45.82,28.4 45.82,33.27 43.69,35.41 39.73,35.41 38.2,36.93 38.2,37.08 37.74,37.54 36.37,37.54 35.31,38.61 35.31,41.27 19.56,57.02 19.56,64.01 | 10.46,63.91 J1.C22 10.44,64.01 19.56,64.01 | JP8.1 17.47,74.12 19.56,72.03 19.56,64.01
GPO_8
  Top 0.152: T9.C 48.56,27.18 48.56,30.68 46.13,33.12 46.13,39.06 37.44,47.75 37.44,62.38 10.46,89.36 J1.C32
GPO_13  (via drill 0.25)
  Top 0.152: v48.72,25.81 48.72,22.15 T10.C | v49.33,31.29 49.63,31.6 49.63,51.71 10.92,90.42 9.85,90.42 8.94,89.51 8.94,87.99 7.87,86.92 J1.B31
  Bottom 0.152: v48.72,25.81 48.72,30.68 v49.33,31.29
IN3  (via drill 0.25)
  Top 0.152: T3.C 40.4,36.39 R38.2 43.54,36.32 v44.45,35.41 | 75.69,31.75 U3.23 75.7,31.75 77.22,31.75 v77.72,32.26 | 110.13,10.39 v110.13,10.41 110.39,10.16 143.76,10.16 145.67,12.06 145.67,17.65 148.18,20.17 148.18,22.61 148.39,22.61 R49.2
  Bottom 0.152: v44.45,35.41 72.19,35.41 75.34,32.26 v77.72,32.26 88.29,32.26 v110.13,10.41
IN4  (via drill 0.25)
  Top 0.152: T4.C 40.4,31.31 R39.2 43.54,31.44 v45.21,33.12 | v74.62,32.21 74.93,32.51 75.54,32.51 U3.24 | R50.2 148.39,25.2 148.13,25.2 145.03,22.1 145.03,12.7 143.26,10.92 91.82,10.92 89.15,13.59 89.15,18.24 84.94,22.45 v84.81,22.45
  Bottom 0.152: 72.64,32.21 72.62,32.21 73.51,31.29 82.35,22.45 v84.81,22.45 | 72.64,32.21 v74.62,32.21 | 72.64,32.21 71.58,33.27 45.36,33.27 v45.21,33.12
IN7  (via drill 0.25)
  Top 0.152: T5.C 40.4,26.23 R40.2 43.54,26.26 v45.21,27.94 | 74.17,33.88 74.17,33.43 73.1,32.36 v71.73,32.36 | 74.17,33.88 U3.25 74.32,34.04 | v116.61,11.4 142.34,11.4 144.4,13.46 144.4,23.68 R51.2 148.39,27.79 | v93.52,34.49 91.24,34.49 88.49,37.24 75.84,37.24 74.17,35.56 74.17,33.88
  Bottom 0.152: v71.73,32.36 71.12,32.97 50.24,32.97 v45.21,27.94 | v93.52,34.49 v116.61,11.4
IN10  (via drill 0.25)
  Top 0.152: T6.C 40.4,21.15 R41.2 43.54,21.23 v44.6,22.3 57.12,8.25 148.28,8.25 149.45,9.42 149.45,28.7 148.54,29.62 148.54,30.23 R52.2 | 73.25,33.88 U3.26 73.37,33.42 v72.8,32.84
  Bottom 0.152: v72.8,32.84 72.47,32.84 71.58,33.73 45.06,33.73 43.33,32 43.43,23.37 44.5,22.3 v44.6,22.3
INHIBIT
  Top 0.152: R48.2 96.08,76.45 99.31,76.45 100.92,74.85 T12.C 100.92,73.83 101.85,72.9 108.2,72.9 108.97,73.66 109.98,73.66 109.98,72.41 U1.34
INHIBIT_R  (via drill 0.25)
  Top 0.152: v96.77,75.06 97.09,75.12 T12.B | JP8.2 17.4,69.09 16.13,67.82 9.14,67.82 7.87,66.55 J1.B23
  Bottom 0.152: JP8.2 77.09,71.63 80.52,75.06 v96.77,75.06
LED_COS
  Top 0.152: U1.56 141.48,77.72 143,76.2 143,72.39 144.27,71.12 R31.2
LED_DMR
  Top 0.152: U1.57 145.54,78.23 147.57,76.2 R33.2
LED_DSTAR
  Top 0.152: U1.58 R34.2
LED_HB
  Top 0.152: U1.55 141.48,77.22 142.49,76.2 142.49,69.85 143.76,68.58 R30.2
LED_NXDN
  Top 0.152: U1.62 118.95,80.77 141.99,80.77 147.57,86.36 R37.2
LED_P25
  Top 0.152: U1.61 118.92,80.26 144.27,80.26 147.57,83.82 R36.2
LED_YSF
  Top 0.152: U1.59 118.92,79.25 145.54,79.25 147.57,81.28 R35.2
LOAD
  Top 0.152: R13.1 R14.1 136.14,68.14 R16.1 145.35,58.29 JP9.1
MISO
  Top 0.152: U3.16 74.17,25.35 74.17,22.3 70.21,18.34 J2.1
  Bottom 0.152: J2.1 69.9,18.49 69.8,18.49 69.34,18.03 13.21,17.98 11.63,19.56 9.65,19.56 9.14,20.07 9.14,27.18 7.9,28.42 J1.B8
MOSI  (via drill 0.25)
  Top 0.152: 68.83,19.05 73.25,23.34 73.25,25.35 U3.15 | 68.83,19.05 68.83,15.29 69.6,14.53 70.97,14.53 72.19,15.75 J2.4 | J1.A7 5.36,25.88 6.6,24.64 6.6,20.07 7.11,19.56 v12.95,19.56 | v67.94,19.05 68.83,19.05
  Bottom 0.152: v12.95,19.56 13.46,19.05 v67.94,19.05
N$1
  Top 0.152: C23.1 123.76,70.68 125.35,69.09 131.52,69.09 OS1.3
N$2
  Top 0.152: R1.2 C2.2
N$4
  Top 0.152: R56.1 LED16.A
N$5
  Top 0.152: R7.1 67.62,85.98 C4.1
N$7
  pour Top: -0.03,100 0.03,97.03 -0.03,97.03
N$8
  Top 0.152: R49.1 LED12.A
N$10
  Top 0.152: IC1.7 IC1.6 89.59,86.61 90.93,86.61 91.19,86.36 91.19,84.33 88.65,81.79 C8.2 87.7,79.25 76.2,79.25 74.8,80.65 C15.2
N$11
  Top 0.152: U1.5 115.06,83.62 115.06,86.99 116.2,88.14 C11.1 116.27,88.58 117.09,89.41 117.09,91.46 Y1.3
N$12
  Top 0.152: U1.6 114.55,83.62 114.55,86.99 113.41,88.14 C9.1 113.09,90.78 Y1.1
N$13
  Top 0.152: R57.1 LED17.A
N$14
  Top 0.152: R50.1 LED13.A
N$15
  Top 0.152: R58.1 LED18.A
N$16
  Top 0.152: R51.1 LED14.A
N$17
  Top 0.152: R5.2 94.05,90.42 87.88,90.42 86.49,89.03 IC1.1 | IC1.1 IC1.2 | TP5.MP 81.15,89.03 IC1.1
N$18
  Top 0.152: R59.1 LED19.A
N$19  (via drill 0.25)
  Top 0.152: R10.2 R9.2 71.95,85.53 v71.88,85.6 | TP2.MP 58.36,90.62 IC2.1 58.49,79.25 v60.2,79.25 | v69.98,76.2 71.31,74.86 R20.1
  Bottom 0.152: v60.2,79.25 63.25,76.2 v69.98,76.2 69.98,81.03 71.88,82.93 v71.88,85.6
N$20
  Top 0.152: R52.1 LED15.A
N$21
  Top 0.152: R9.1 72.96,83.57 69.6,83.57 68.65,83.63 R7.2 64.96,80.52 62.74,80.52 60.07,77.85 IC2.2 58.23,77.98 57.15,77.98 55.37,79.76 55.37,88.39 53.59,90.17 TP1.MP
N$24
  Top 0.152: R8.2 C8.1 88.71,78.23 90.17,78.23 92.2,80.26 92.2,82.8 93.03,83.63 R6.1
N$25
  Top 0.152: IC1.5 89.15,84.9 89.15,84.07 85.28,80.2 R8.1 C10.1
N$26
  Top 0.152: R5.1 R6.2 94.3,85.6 95.25,85.6 97.22,83.63 C3.1
N$28
  Top 0.152: C2.1 53.34,76.45 | 53.34,76.45 R4.1 | IC2.3 58.23,76.45 53.34,76.45
N$29
  Top 0.152: R2.2 53.41,67.31 | 53.41,67.31 54.36,67.31 55.37,68.33 55.37,70.36 | 55.37,70.36 55.37,71.63 54.04,72.96 R4.2 | C1.1 58.04,70.36 55.37,70.36 | 53.41,67.31 53.34,67.24 R3.2
N$30
  Top 0.152: R28.1 LED2.A
N$33
  Top 0.152: R29.1 LED3.A
N$34
  Top 0.152: R30.1 LED4.A
N$38
  Top 0.152: R29.2 143.76,88.9 137.99,83.13 T2.C
N$40
  Top 0.152: R33.1 LED7.A
N$41
  Top 0.152: C14.1 64.26,67.38 | R15.2 63.31,62.23 64.01,62.23 64.26,62.48 64.26,67.38 | 64.26,67.38 R12.1
N$42
  Top 0.152: R15.1 61.98,64.2 | 61.98,64.2 C16.1 | IC2.5 63.43,75.44 62.48,75.44 61.98,74.93 61.98,64.2
N$43  (via drill 0.25)
  Top 0.152: R12.2 C12.1 69.02,73.91 74.68,73.91 76.2,75.44 v76.2,78.23 | v76.2,80.77 78.99,83.57 R10.1
  Bottom 0.152: v76.2,78.23 v76.2,80.77
N$44
  Top 0.152: R34.1 LED8.A
N$45
  Top 0.152: R35.1 LED9.A
N$46
  Top 0.152: R36.1 LED10.A
N$51
  Top 0.152: R31.1 LED5.A
N$52
  Top 0.152: R32.1 LED6.A
N$54
  Top 0.152: IC3.6 84.01,71.12 88.65,71.12 | 88.65,71.12 R21.2 | R22.1 88.65,71.12
N$55  (via drill 0.25)
  Top 0.152: R23.1 88.65,64.45 R22.2 88.58,67.31 v83.31,67.31 | v81.28,67.31 81.28,70.36 80.64,70.99 IC3.3
  Bottom 0.152: v83.31,67.31 v81.28,67.31
N$56
  Top 0.406: LED4.C LED5.C LED6.C LED7.C LED8.C LED9.C LED10.C LED11.C LED3.C LED2.C 154.94,91.47 154.94,92.46 153.92,93.47 142.24,93.47 139.95,91.19 JP1.1
N$57
  Top 0.152: LED1.A R25.1
N$58  (via drill 0.25)
  Top 0.152: LED1.C 152.69,64.01 v150.11,64.01 | T1.C 73.66,63.18 73.66,61.98 75.18,60.58 v118.87,60.58
  Bottom 0.152: v150.11,64.01 122.3,64.01 v118.87,60.58
N$59  (via drill 0.25)
  Top 0.152: R20.2 74.36,72.26 IC3.2 v80.9,72.26 | v85.98,69.72 IC3.5
  Bottom 0.152: v80.9,72.26 83.44,69.72 v85.98,69.72
N$60
  Top 0.152: IC3.7 83.75,72.14 82.3,72.14 82.3,67.06 83.14,66.21 D1.2
N$61  (via drill 0.25)
  Top 0.152: IC3.1 80.9,73.53 81.91,72.52 v81.91,66.04 | v81.91,61.59 82.62,62.3 D1.1
  Bottom 0.152: v81.91,66.04 v81.91,61.59
N$63
  Top 0.152: D1.3 77.08,63.25 T1.B 74.93,63.5 74.93,66.11 C22.1
N$65
  Top 0.152: R37.1 LED11.A
NRST  (via drill 0.25)
  Top 0.152: v107.44,68.83 112.27,68.83 113.28,67.82 JP3.6 112.01,65.28 112.01,63.25 112.52,62.74 122.68,62.74 124.71,60.71 R17.2 126.3,60.51 127.89,58.93 129.48,58.93 R11.2 129.79,58.93 131.06,58.93 132.65,60.51 C13.1 134.56,60.83 139.95,60.83 142.49,58.29 142.49,55.75 JP10.1 | v114.05,81.53 U1.7
  Bottom 0.152: v107.44,68.83 107.44,73.15 108.2,73.91 112.27,73.91 114.05,75.69 v114.05,81.53
OPTID
  Top 0.152: J1.C19 11.09,55.69 R55.2 R54.1
OPTIRQ  (via drill 0.25)
  Top 0.152: v64.95,16.99 70.97,23.01 70.97,25.35 U3.12
  Bottom 0.152: J1.A25 2.54,68.81 2.54,34.42 4.7,32.26 5.59,32.26 6.6,31.24 6.6,17.91 7.44,17.02 63.7,17.02 v64.95,16.99
OUT0  (via drill 0.25)
  Top 0.152: T7.B 51,36.32 55.73,31.6 67,31.6 U3.2 67.16,31.6 68.33,31.6 v68.99,30.94 | R56.2 146.5,8.64 83.69,8.64 78.99,13.33 v78.99,19.56
  Bottom 0.152: v68.99,30.94 68.99,29.92 69.6,29.31 v78.99,19.56
OUT2  (via drill 0.25)
  Top 0.152: v67.56,25.5 68.53,25.5 U3.9 | v63.42,29.77 52.53,29.77 51,31.29 T8.B | R57.2 148.34,13.21 147.32,12.19 147.32,10.54 145.8,9.02 84.2,9.02 v83.69,9.52
  Bottom 0.152: v63.42,29.77 v67.56,25.5 67.72,25.5 v83.69,9.52
OUT8  (via drill 0.25)
  Top 0.152: T9.B 51,26.11 54.41,22.71 67.11,22.71 69.29,24.89 69.29,25.35 U3.10 69.44,25.5 69.44,25.96 69.42,25.98 v69.42,27.08 | R58.2 146.81,14.03 146.81,11.18 145.03,9.4 87.25,9.4 v85.19,11.43
  Bottom 0.152: v69.42,27.08 69.57,27.08 69.72,26.92 v85.19,11.43
OUT13  (via drill 0.25)
  Top 0.152: 70.05,25.35 U3.11 70.21,25.39 v70.21,24.28 67.16,21.23 51,21.23 T10.B | 148.39,18.19 R59.2 146.3,16.06 146.3,11.68 144.4,9.78 88.65,9.78 v87.76,10.67
  Bottom 0.152: v87.76,10.67 83.82,10.67 v70.21,24.28
PTT  (via drill 0.25)
  Top 0.152: T11.B 101.71,72.36 U1.33 109.52,70.79 v109.6,70.74 | R32.2 v143.76,73.66
  Bottom 0.152: v143.76,73.66 142.24,71.63 115.57,71.63 114.68,70.74 v109.6,70.74
PTT_R  (via drill 0.25)
  Top 0.152: T11.C 102.42,69.72 v102.49,69.72 | 14.86,72.9 17.65,72.9 18.92,71.63 v18.92,70.36 | J1.A23 5.33,66.55 7.85,69.06 J1.B24 7.87,69.09 9.14,70.36 9.14,72.14 9.91,72.9 14.86,72.9 | JP8.4 14.86,72.9
  Bottom 0.152: v102.49,69.72 101.22,68.45 83.44,68.45 81.53,70.36 v18.92,70.36
RESET
  Top 0.152: U2.A12 132.33,44.96 130.68,46.61 125.98,46.61 124.71,47.88 R17.1 121.22,58.61 120.9,58.29 112.65,58.29 110.74,56.39 JP5.4
RSSI  (via drill 0.25)
  Top 0.152: TP7.MP 92.71,64.26 92.71,68.07 93.91,69.28 C30.2 R53.2 96.07,72.96 v96.14,72.9 | U1.27 107.64,76.71 106.55,76.71 v105.92,76.07
  Bottom 0.152: v105.92,76.07 99.31,76.07 v96.14,72.9
RSSI_R  (via drill 0.25)
  Top 0.152: R53.1 94.23,76.07 93.85,76.45 78.99,76.45 v78.61,76.07 | J1.A22 5.33,64.01 4.06,65.28 4.06,74.93 4.57,75.44 v13.59,75.44
  Bottom 0.152: v78.61,76.07 78.36,76.07 77.72,75.44 v13.59,75.44
RST  (via drill 0.25)
  Top 0.152: R24.2 70.37,37.4 | 70.37,37.4 70.97,36.79 U3.29 70.97,33.88 v70.97,32.36 | 79.65,21.08 82.09,21.08 C18.1 | 79.65,21.08 72.95,14.38 71.27,14.38 J2.5 | 70.37,37.4 72.8,39.83 86.36,39.83 90.47,35.71 94.74,35.71 D2.3 | 70.36,37.39 70.37,37.4 | v79.65,22.3 79.65,21.08
  Bottom 0.152: v79.65,22.3 70.97,30.99 v70.97,32.36
RXA  (via drill 0.25)
  Top 0.152: 65.4,76.58 65.4,71.44 C14.2 64.2,68.33 69.09,68.33 69.6,67.82 69.6,64.77 TP3.MP | 65.4,76.58 IC2.6 IC2.7 | U1.26 v105.92,77.22 | v71.25,77.22 69.21,79.25 66.29,79.25 65.4,78.49 65.4,76.58
  Bottom 0.152: v105.92,77.22 v71.25,77.22
RXA_R  (via drill 0.25)
  Top 0.152: v46.61,83.06 48.26,83.06 50.73,85.53 R1.1
  Bottom 0.152: J1.A16 6.6,50.01 6.6,82.3 7.37,83.06 v46.61,83.06
RXD_HOST  (via drill 0.25)
  Top 0.152: U1.43 114.55,72.34 114.55,69.6 115.82,68.33 v115.82,65.79 | JP5.2 115.82,48.13 118.36,45.59 126.62,45.59 127.25,44.96 U2.A8 | U2.A8
  Bottom 0.152: v115.82,65.79 JP5.2
RXI
  Top 0.152: U3.30 70.21,33.88 70.21,32.36 70.81,31.75 73.41,31.75 76.45,34.8 88.34,34.8 89.1,34.04 89.1,29.77 87.88,28.55 J3.TXO
  Bottom 0.152: JP7.4 87.88,20.34 85.95,22.28 85.95,26.52 J3.TXO
SBC_DTR  (via drill 0.25)
  Top 0.152: Q4.2 100.34,30.8 R44.2 104.58,30.8 v105.66,29.72 | U2.A24 146.3,42.77 146.3,26.16 143.76,23.62 143.76,14.35 141.35,11.94 v118.36,11.94
  Bottom 0.152: v118.36,11.94 105.66,24.64 v105.66,29.72
SBC_RX
  Top 0.152: Q2.2 103.58,19.83 R42.2 111.06,12.45 140.84,12.45 143,14.6 143,23.88 143.76,24.64 143.76,42.74 145.06,44.04 U2.A22 | JP6.3 140.59,51.94 145.03,47.5 U2.A22 | U2.A22
SBC_SCL  (via drill 0.25)
  Top 0.152: R19.1 108.9,38.29 109.85,39.24 113.41,39.24 114.66,40.49 v114.66,45.16 114.71,45.21 123.06,45.21 123.44,44.96 123.44,42.77 U2.A5 | v16.13,29.21 12.8,25.88 J1.C7
  Bottom 0.152: v114.66,45.16 114.4,45.16 114.25,45.01 31.95,45.01 16.15,29.21 v16.13,29.21
SBC_SDA  (via drill 0.25)
  Top 0.152: R18.1 113.1,38.29 117.6,42.8 120.87,42.8 U2.A3 | v113.66,45.57 v113.66,42.8 | v16.76,31.5 16.76,24.64 12.93,20.8 J1.C5
  Bottom 0.152: v113.66,45.57 113.64,45.57 113.41,45.34 31.04,45.31 30.58,45.31 v16.76,31.5 | v113.66,42.8 120.87,42.8 U2.A3
SBC_TX
  Top 0.152: Q3.2 100.31,25.34 R43.2 | 103.63,25.15 R43.2 | R43.2 103.73,25.35 104.65,25.35 106.43,27.13 106.43,31.11 115.32,40 130.94,40 132.33,41.4 U2.A11 132.38,41.5 133.6,42.72 133.6,47.9 139.85,54.15 139.85,54.46 JP6.2
SPICLK
  Top 0.152: U3.17 75.54,26.87 75.54,22.91 71.27,18.64 71.27,16.81 70.21,15.75 J2.3
  Bottom 0.152: 10.46,28.4 J1.C8 12.29,26.54 12.29,21.64 13.99,19.94 70.51,19.94 71.27,18.8 71.27,16.81 70.21,15.75 J2.3
STN5V
  Top 0.152: R54.2 17.14,52.96 14.22,50.04 4.83,50.04 3.56,48.77 3.56,16.26 4.06,15.75 5.28,15.75 J1.A3 5.44,15.75 7.87,15.75 | 7.87,15.75 10.31,15.75 J1.C3 | 7.87,15.75 J1.B3
SWCLK  (via drill 0.25)
  Top 0.152: U1.49 118.85,74.17 118.87,74.17 v118.87,70.87
  Bottom 0.152: v118.87,70.87 116.84,68.83 111.51,68.83 110.74,68.07 JP3.4
SWDIO  (via drill 0.25)
  Top 0.152: U1.46 116.08,72.31 v116.08,69.6
  Bottom 0.152: v116.08,69.6 109.22,69.6 108.2,68.58 JP3.2
TXA
  Top 0.152: U1.20 107.64,80.26 106.04,80.26 104.27,82.04 97.79,82.04 95.25,84.58 92.71,84.58 91.95,85.34 91.95,87.63 91.19,88.39 88.14,88.39 86.23,86.49 IC1.3
TXA_R  (via drill 0.25)
  Top 0.152: TP6.MP 71.37,88.9 71.37,85.34 72.14,84.58 74.93,84.58 75.18,84.33 75.18,82.8 74.68,82.3 72.39,82.3 71.88,81.79 71.88,78.74 72.77,77.85 C15.1 | v50.42,84.33 47.88,81.79 v46.61,81.79
  Bottom 0.152: TP6.MP 73.41,89.53 72.64,88.77 54.89,88.77 50.44,84.35 v50.42,84.33 | v46.61,81.79 16.76,81.79 12.95,77.98 12.95,51.28 J1.C16
TXD_HOST  (via drill 0.25)
  Top 0.152: v115.32,74.93 114.05,73.66 U1.42 v114.05,68.33 | v122.94,81.28 129.92,81.28 132.97,84.33 134.24,84.33 134.75,84.84 134.75,85.46 T2.B | JP5.1 118.36,48.13 120.4,46.1 128.65,46.1 129.79,44.96 U2.A10 | U2.A10
  Bottom 0.152: v122.94,81.28 116.59,74.93 v115.32,74.93 | v114.05,68.33 116.59,65.79 116.59,57.4 118.36,55.63 JP5.1
TXO  (via drill 0.25)
  Top 0.152: v74.24,31.44 70.66,31.44 69.44,32.66 69.44,33.88 U3.31
  Bottom 0.152: v74.24,31.44 85.75,31.44 87.43,29.77 88.49,29.77 88.52,29.72 89.15,29.08 89.15,27.18 87.93,25.96 87.88,25.96 J3.RXI 86.36,24.38 86.36,22.99 89.15,20.19 89.15,15.75 JP7.2
VCAP
  Top 0.152: JP12.2 102.74,80.26 102.43,80.2 C7.2
VCAP_1A
  Top 0.152: JP12.3 103.07,79.38 103.76,79.38 104.39,78.74 104.39,76.33 | 104.39,76.33 104.39,75.56 105.28,74.68 107.62,74.68 U1.31 | JP13.1 103.02,76.33 104.39,76.33
VCAP_1B
  Top 0.152: U1.30 107.62,75.18 105.54,75.18 104.9,75.82 104.9,80.39 104.22,81.08 JP12.1
VCAP_2
  Top 0.152: U1.47 116.53,70.92 118.36,69.09 C33.2
VDDA  (via drill 0.25)
  Top 0.152: U1.13 111,83.62 111,84.96 111.38,85.34 v113.28,85.34 | v115.82,85.34 120.74,85.34 L1.2 123.29,86.07 C5.2 C6.2
  Bottom 0.152: v113.28,85.34 v115.82,85.34
XTAL1
  Top 0.152: U3.7 67.05,27.69 64.01,27.69 62.88,26.56 Y2.3 62.78,26.54 60.32,26.54 60.26,26.61 C31.1
XTAL2
  Top 0.152: 66.98,26.92 U3.8 66.92,26.92 66.92,25.52 65.53,24.13 64.66,24.13 Y2.1 | Y2.1 65.02,24.49 | C32.1 61.4,25.27 63.45,25.27 Y2.1
~RESET
  Top 0.152: JP11.1 19.91,48.67 11.84,48.67 10.77,47.6 8.94,47.6 7.87,48.67 J1.B16
~SS  (via drill 0.25)
  Top 0.152: v72.64,27.03 72.64,25.5 U3.14 | v70.18,30.96 67.87,33.27 64.26,33.27 D3.3
  Bottom 0.152: v70.18,30.96 72.64,28.5 v72.64,27.03

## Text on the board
tNames: RX | TX | PWR | ACT | NXD | P25 | YSF | MODEM | D* | STM32F446RET6 | DMR | PTT | MODEM INDICATORS | ANALOG / HANDSHAKE / ENABLE | COS | HB | CLP | Install to / Emulate / Aux I/O Card | CLIP | LOAD | GND | RESET | BOOT | HOST TXD | HOST RXD | WA0EDA | STM32-DVM-MTR2K v2.0c | NanoPi NEO | (C) 2019 THE REGENTS OF THE K0USY GROUP | +V | GND | I/O INDICATORS | <10 | <7 | UART LEVEL SHIFT | <4 | <3 | I/O PROCESSOR | Licensed under CC BY-NC-SA 4.0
